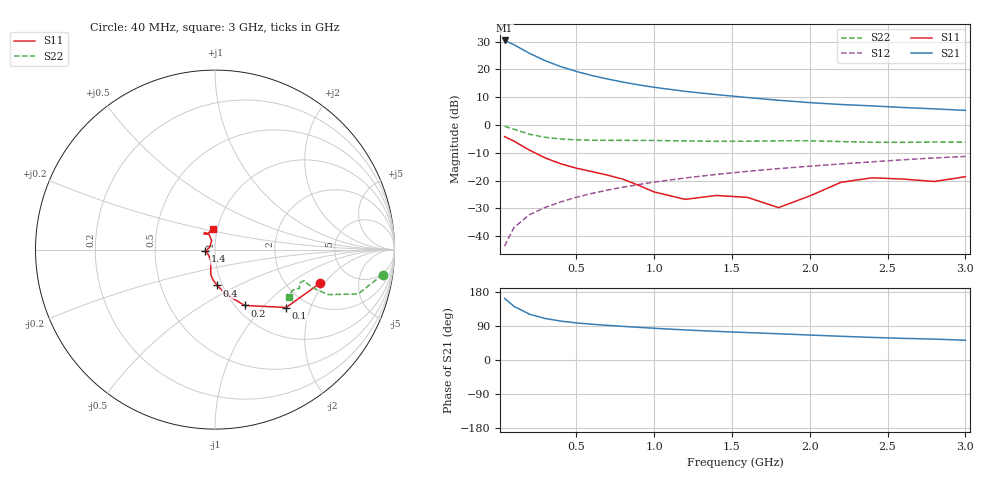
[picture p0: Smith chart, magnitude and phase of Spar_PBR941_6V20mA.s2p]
! Filename:  PBR941P.S2P  Version:  3.0
! NXP part #:  PBR941  Date: July 1998
! Bias condition:  Vce=6V, Ic=20mA
#  MHz  S  MA  R 50
! Freq  S11  S21  S12  S22
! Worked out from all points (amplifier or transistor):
!   21 points, 40 MHz to 3 GHz, reference 50 ohm
!   highest |S21| = 30.4 dB at 40 MHz (marker M1)
!   |S21| within 3 dB of that: start of sweep to 147.2 MHz
!   unconditionally stable (mu >= 1): 782.3 MHz to 2.239 GHz
!   at 300 MHz: K = 0.84, MSG = 26.4 dB, |S12| = -29.7 dB
!   at 1 GHz: K = 1.02, MAG = 16.2 dB, |S12| = -20.6 dB
!   at 3 GHz: K = 0.98, MSG = 8.3 dB, |S12| = -11.3 dB
!   lowest NFmin = 2.27 dB at 500 MHz
!   S11 on the Smith chart (normalised r, x): 40 MHz: 3.03, -1.81; 100 MHz: 1.58, -1.38; 200 MHz: 1.10, -0.78; 400 MHz: 0.94, -0.39; 1.4 GHz: 0.90, -0.02; 3 GHz: 0.95, +0.22
40  0.616 -17.5  33.04 162.5  0.006603 81.1  0.9451 -8.4
100  0.5113 -39.1  27.68 141.7  0.01426 76.2  0.8349 -17.2
200  0.3519 -62.1  19.38 120.8  0.02437 72.7  0.6797 -21.6
300  0.2554 -76.4  14.32 109.6  0.03277 74.1  0.5995 -21.4
400  0.2003 -86.5  11.19 102.7  0.04124 75.7  0.559 -20.6
500  0.1669 -94.2  9.175 97.9  0.04988 77.0  0.5393 -20.0
600  0.1451 -98.7  7.752 94.4  0.05859 77.7  0.5305 -19.6
700  0.1255 -101.0  6.702 91.5  0.06721 78.5  0.5276 -19.4
800  0.1057 -103.0  5.892 88.8  0.07584 79.1  0.528 -19.3
900  0.08236 -106.4  5.255 86.2  0.0847 79.0  0.527 -19.3
1000  0.06245 -113.1  4.755 83.8  0.09367 79.4  0.5255 -19.4
1200  0.04588 -149.0  4.014 79.3  0.1113 79.1  0.5164 -20.1
1400  0.05393 -170.6  3.509 75.6  0.1289 78.6  0.507 -21.7
1600  0.04976 -172.0  3.11 72.4  0.1464 78.4  0.5092 -23.2
1800  0.03256 156.7  2.776 69.3  0.1639 78.1  0.518 -24.2
2000  0.0528 110.5  2.519 65.9  0.181 77.2  0.5173 -24.8
2200  0.09269 111.1  2.331 62.6  0.199 76.3  0.5021 -25.6
2400  0.112 121.3  2.198 59.6  0.2169 75.5  0.4878 -27.7
2600  0.1063 125.3  2.058 57.2  0.2361 75.1  0.4857 -30.4
2800  0.09608 115.2  1.944 55.1  0.2549 74.4  0.4926 -32.3
3000  0.1172 96.5  1.825 52.1  0.2715 73.2  0.4896 -32.8
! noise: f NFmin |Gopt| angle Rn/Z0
500  2.273  0.074  29.79  0.237
900  2.274  0.03  -135.1  0.187
1000  2.332  0.017  26.68  0.255
2000  2.913  0.178  -121.3  0.337
